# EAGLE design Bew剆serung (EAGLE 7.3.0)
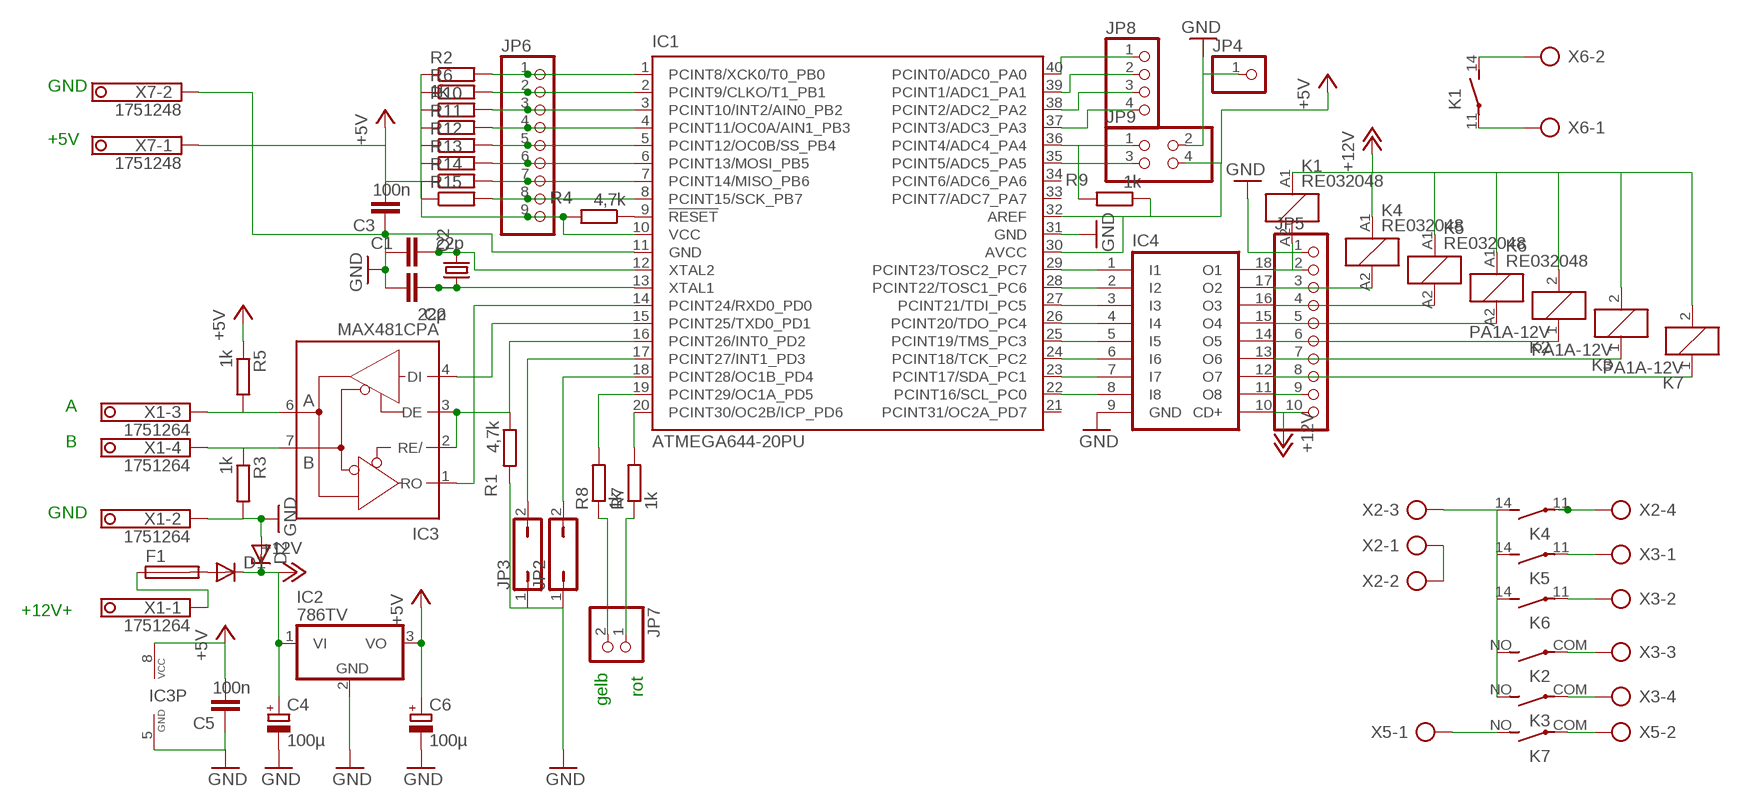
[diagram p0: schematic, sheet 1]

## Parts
C1  22p  C-EUC0603  [C0603]
C2  22p  C-EUC0603  [C0603]
C3  100n  C-EUC1206  [C1206]
C4  100µ  CPOL-EUSMCD  [SMC_D]
C5  100n  C-EU050-024X044  [C050-024X044]
C6  100µ  CPOL-EUSMCD  [SMC_D]
D1  DIODE-DO214AA  [DO214AA]
D2  ZENER-DIODESOD80C  [SOD80C]
F1  19560  [19560]
IC1  ATMEGA644-20PU  [DIL40]
IC2  786TV  [TO220V]
IC3  MAX481CPA  [DIL08]
IC4  ULN2803A  [DIL18]
JP2  JP1Q  [JP1]
JP3  JP1Q  [JP1]
JP4  PINHD-1X1  [1X01]
JP5  PINHD-1X10  [1X10]
JP6  PINHD-1X9  [1X09]
JP7  PINHD-1X2  [1X02]
JP8  PINHD-1X4  [1X04]
JP9  PINHD-2X2  [2X02]
K1  RE032048  [RE-SCHRACK]
K2  PA1A-12V  [PA]
K3  PA1A-12V  [PA]
K4  RE032048  [RE-SCHRACK]
K5  RE032048  [RE-SCHRACK]
K6  RE032048  [RE-SCHRACK]
K7  PA1A-12V  [PA]
Q2  CRYSTALCTS406  [CTS406]
R1  4,7k  R-EU_R0603  [R0603]
R2  1k  R-EU_R0603  [R0603]
R3  1k  R-EU_R1206  [R1206]
R4  4,7k  R-EU_R0603  [R0603]
R5  1k  R-EU_R1206  [R1206]
R6  R-EU_R0603  [R0603]
R7  1k  R-EU_R0603  [R0603]
R8  1k  R-EU_R0603  [R0603]
R9  1k  R-EU_R0603  [R0603]
R10  R-EU_R0603  [R0603]
R11  R-EU_R0603  [R0603]
R12  R-EU_R0603  [R0603]
R13  R-EU_R0603  [R0603]
R14  R-EU_R0603  [R0603]
R15  R-EU_R0603  [R0603]
X1  1751264  [1751264]
X2  AK300/4  [AK300/4]
X3  AK300/4  [AK300/4]
X5  AK300/2  [AK300/2]
X6  AK300/2  [AK300/2]
X7  1751248  [1751248]

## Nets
+5V: C3.2 C5.2 C6.+ IC1.10(VCC) IC1.30(AVCC) IC1.32(AREF) IC2.3(VO) IC3.8(VCC) JP6.9 JP9.4 R2.1 R4.2 R5.1 R6.1 R9.1 R10.1 R11.1 R12.1 R13.1 R14.1 R15.1 X7.1
+12V: C4.+ D1.C D2.C IC2.1(VI) IC4.10(CD+) JP5.10 K1.A1 K2.2 K3.2 K4.A1 K5.A1 K6.A1 K7.2
GND: C1.1 C2.1 C3.1 C4.- C5.1 C6.- D2.A IC1.11(GND) IC1.31(GND) IC2.2(GND) IC3.5(GND) IC4.9(GND) JP2.1 JP3.1 JP4.1 JP5.1 JP9.2 R1.2 R3.2 X1.2 X7.2
N$1: D1.A F1.2
N$2: IC1.14(PCINT24/RXD0_PD0) IC3.1(RO)
N$3: IC3.7(B) R3.1 X1.4
N$4: IC3.6(A) R5.2 X1.3
N$5: IC4.18(O1) JP5.2 K1.A2
N$6: IC1.2(PCINT9/CLKO/T1_PB1) JP6.2 R6.2
N$7: IC1.40(PCINT0/ADC0_PA0) JP8.1
N$8: K4.11(2:P) X2.4
N$9: IC1.29(PCINT23/TOSC2_PC7) IC4.1(I1)
N$10: IC1.15(PCINT25/TXD0_PD1) IC3.4(DI)
N$11: C2.2 IC1.13(XTAL1) Q2.1
N$12: C1.2 IC1.12(XTAL2) Q2.3
N$13: IC1.16(PCINT26/INT0_PD2) IC3.2(RE/) IC3.3(DE) R1.1
N$14: IC1.17(PCINT27/INT1_PD3) JP3.2
N$15: IC1.18(PCINT28/OC1B_PD4) JP2.2
N$16: IC1.28(PCINT22/TOSC1_PC6) IC4.2(I2)
N$17: IC1.27(PCINT21/TDI_PC5) IC4.3(I3)
N$18: IC1.26(PCINT20/TDO_PC4) IC4.4(I4)
N$19: IC1.19(PCINT29/OC1A_PD5) R8.2
N$20: IC1.9(!RESET) R4.1
N$21: IC1.20(PCINT30/OC2B/ICP_PD6) R7.2
N$22: JP7.2 R8.1
N$23: IC1.25(PCINT19/TMS_PC3) IC4.5(I5)
N$24: IC1.24(PCINT18/TCK_PC2) IC4.6(I6)
N$25: JP7.1 R7.1
N$26: IC1.23(PCINT17/SDA_PC1) IC4.7(I7)
N$27: IC1.22(PCINT16/SCL_PC0) IC4.8(I8)
N$28: IC4.17(O2) JP5.3 K4.A2
N$29: IC4.16(O3) JP5.4 K5.A2
N$30: IC4.15(O4) JP5.5 K6.A2
N$31: IC4.14(O5) JP5.6 K2.1
N$32: IC4.13(O6) JP5.7 K3.1
N$33: K1.14(2:S) X6.2
N$34: K1.11(2:P) X6.1
N$35: K2.NO(2:S) K3.NO(2:S) K4.14(2:S) K5.14(2:S) K6.14(2:S) X2.3
N$36: IC1.39(PCINT1/ADC1_PA1) JP8.2
N$37: IC1.38(PCINT2/ADC2_PA2) JP8.3
N$38: IC1.37(PCINT3/ADC3_PA3) JP8.4
N$39: IC1.36(PCINT4/ADC4_PA4) JP9.1 R9.2
N$40: IC1.35(PCINT5/ADC5_PA5) JP9.3
N$41: K5.11(2:P) X3.1
N$42: K6.11(2:P) X3.2
N$43: K2.COM(2:P) X3.3
N$44: K3.COM(2:P) X3.4
N$45: K7.COM(2:P) X5.2
N$46: F1.1 X1.1
N$47: IC1.8(PCINT15/SCK_PB7) JP6.8 R15.2
N$48: IC1.7(PCINT14/MISO_PB6) JP6.7 R14.2
N$49: IC1.6(PCINT13/MOSI_PB5) JP6.6 R13.2
N$50: IC1.5(PCINT12/OC0B/SS_PB4) JP6.5 R12.2
N$51: IC1.4(PCINT11/OC0A/AIN1_PB3) JP6.4 R11.2
N$52: IC1.3(PCINT10/INT2/AIN0_PB2) JP6.3 R10.2
N$53: IC1.1(PCINT8/XCK0/T0_PB0) JP6.1 R2.2
N$54: K7.NO(2:S) X5.1
N$55: IC4.12(O7) JP5.8 K7.1
N$56: IC4.11(O8) JP5.9
N$60: X2.1 X2.2
Unconnected: IC1.21(PCINT31/OC2A_PD7) IC1.33(PCINT7/ADC7_PA7) IC1.34(PCINT6/ADC6_PA6)

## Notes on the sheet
- GND
- +5V
- A
- B
- GND
- +12V+
- rot
- gelb

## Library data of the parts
C1-C3 C5 = rcl:C-EU: CAPACITOR, European symbol
C4 C6 = rcl:CPOL-EU: POLARIZED CAPACITOR, European symbol
D1 = diode:DIODE-: DIODE
D2 = diode:ZENER-DIODE: Z-Diode
F1 = fuse:19560: FUSE HOLDER; MPN: 56000001009; OC_FARNELL: 1185363; OC_NEWARK: 15P8392
IC1 = atmel:ATMEGA644-*PU: 8-bit Microcontroller with 64K Bytes In-System Programmable Flash Auto generated by make-symbol-device-package-bsdl.ulp Rev. 34 Source: http://www.atmel.com/dyn/resources/prod_documents/doc2593.pdf; MPN: ATMEGA644-20PU; OC_FARNELL: 1288340; OC_NEWARK: 23M5060
IC2 = linear:78*: Positive VOLTAGE REGULATOR Source: http://cache.national.com/ds/LM/LM78L05.pdf http://www.fairchildsemi.com/ds/LM/LM7805.pdf
IC3 = maxim:MAX481CPA: RS485 TRANSEIVER; MPN: MAX481CPA+; OC_FARNELL: unknown; OC_NEWARK: 99K3445
IC4 = uln-udn:ULN2803A: DRIVER ARRAY
JP2 JP3 = jumper:JP1Q: JUMPER
JP4 = pinhead:PINHD-1X1: PIN HEADER
JP5 = pinhead:PINHD-1X10: PIN HEADER
JP6 = pinhead:PINHD-1X9: PIN HEADER
JP7 = pinhead:PINHD-1X2: PIN HEADER
JP8 = pinhead:PINHD-1X4: PIN HEADER
JP9 = pinhead:PINHD-2X2: PIN HEADER
K1 K4-K6 = relay:RE03*: Miniature PCB Relay 1 pole 6 A SCHRACK Source: http://www.schrack.com/.. 5812.pdf; OC_FARNELL: unknown; OC_NEWARK: unknown
K2 K3 K7 = relay:PA?*: SLIM POWER RELAY NAiS Source: http://www.mew-europe.com/.. en_ds_61123_0000.pdf; MF: AROMAT/ MATSUSHITA; MPN: PA1A-12V-Y1; OC_FARNELL: 910363; OC_NEWARK: 82H8374
Q2 = crystal:CRYSTAL: CRYSTAL; OC_FARNELL: unknown; OC_NEWARK: unknown
R1-R15 = rcl:R-EU_: RESISTOR, European symbol
X1 = con-phoenix-350:1751264: MKDS 1/ 4-3,5 Printklemme Nennstrom: 10 A Bemessungsspannung: 160 V Raster: 3,5 mm Polzahl: 4 Montageart: Löten Anschlussart: Schraubanschluss Anschlussrichtung vom Leiter zur Platine: 0° Source: http://eshop.phoenixcontact.com .. 1751264.pdf
X2 X3 = con-ptr500:AK300/4: CONNECTOR; OC_FARNELL: unknown; OC_NEWARK: unknown
X5 X6 = con-ptr500:AK300/2: CONNECTOR; OC_FARNELL: unknown; OC_NEWARK: unknown
X7 = con-phoenix-350:1751248: MKDS 1/ 2-3,5 Printklemme

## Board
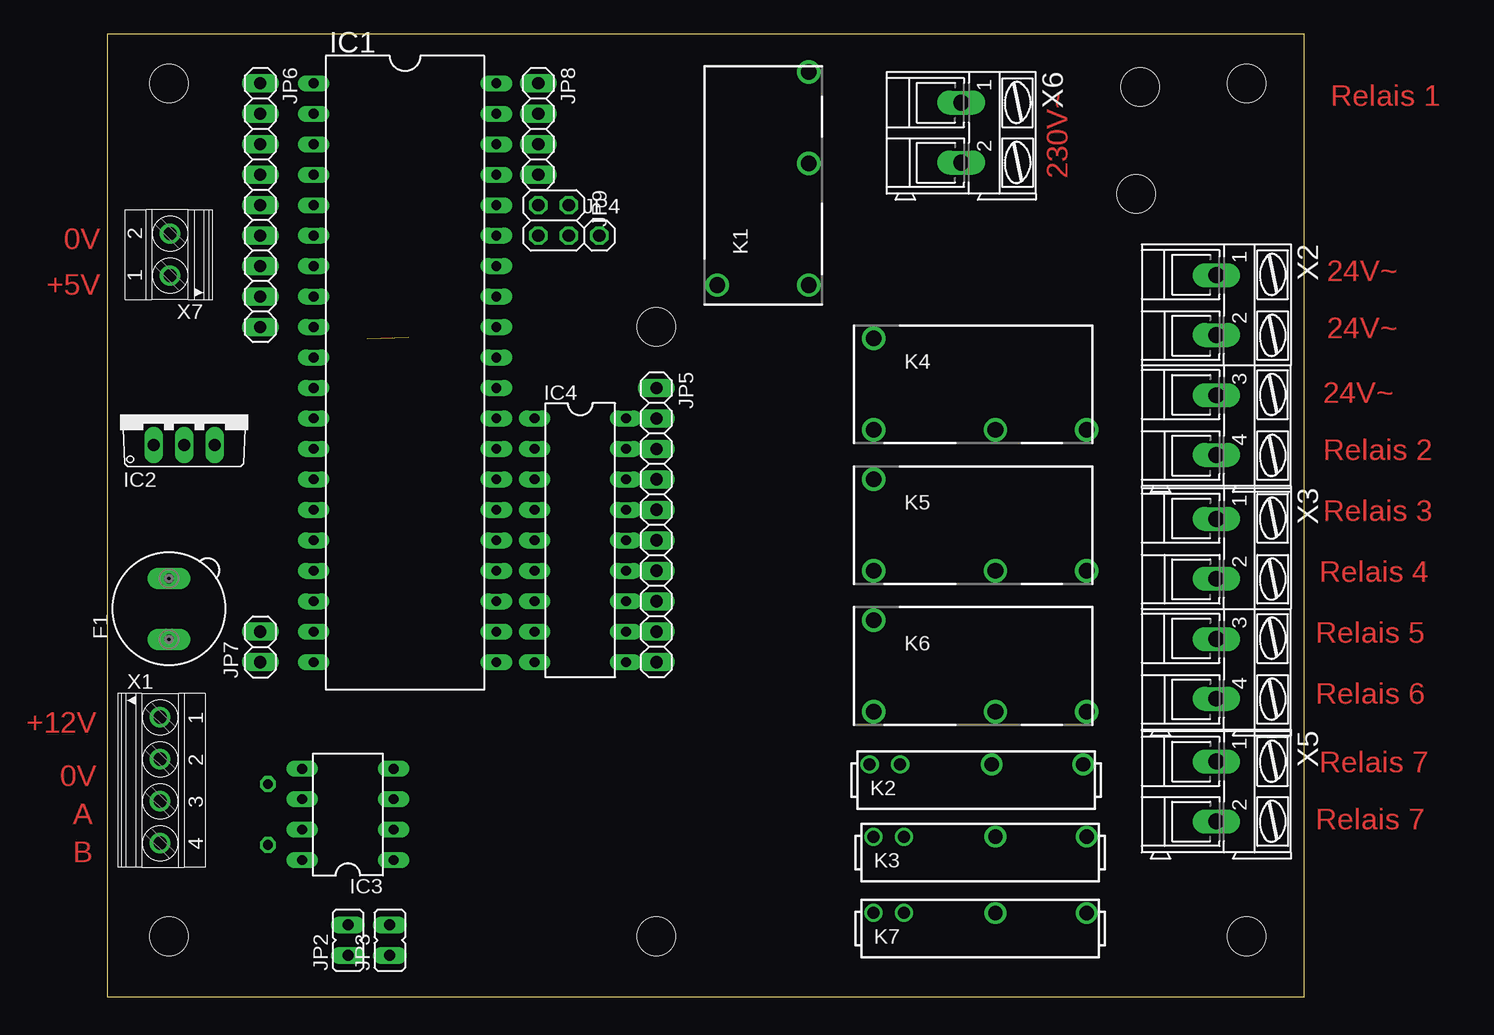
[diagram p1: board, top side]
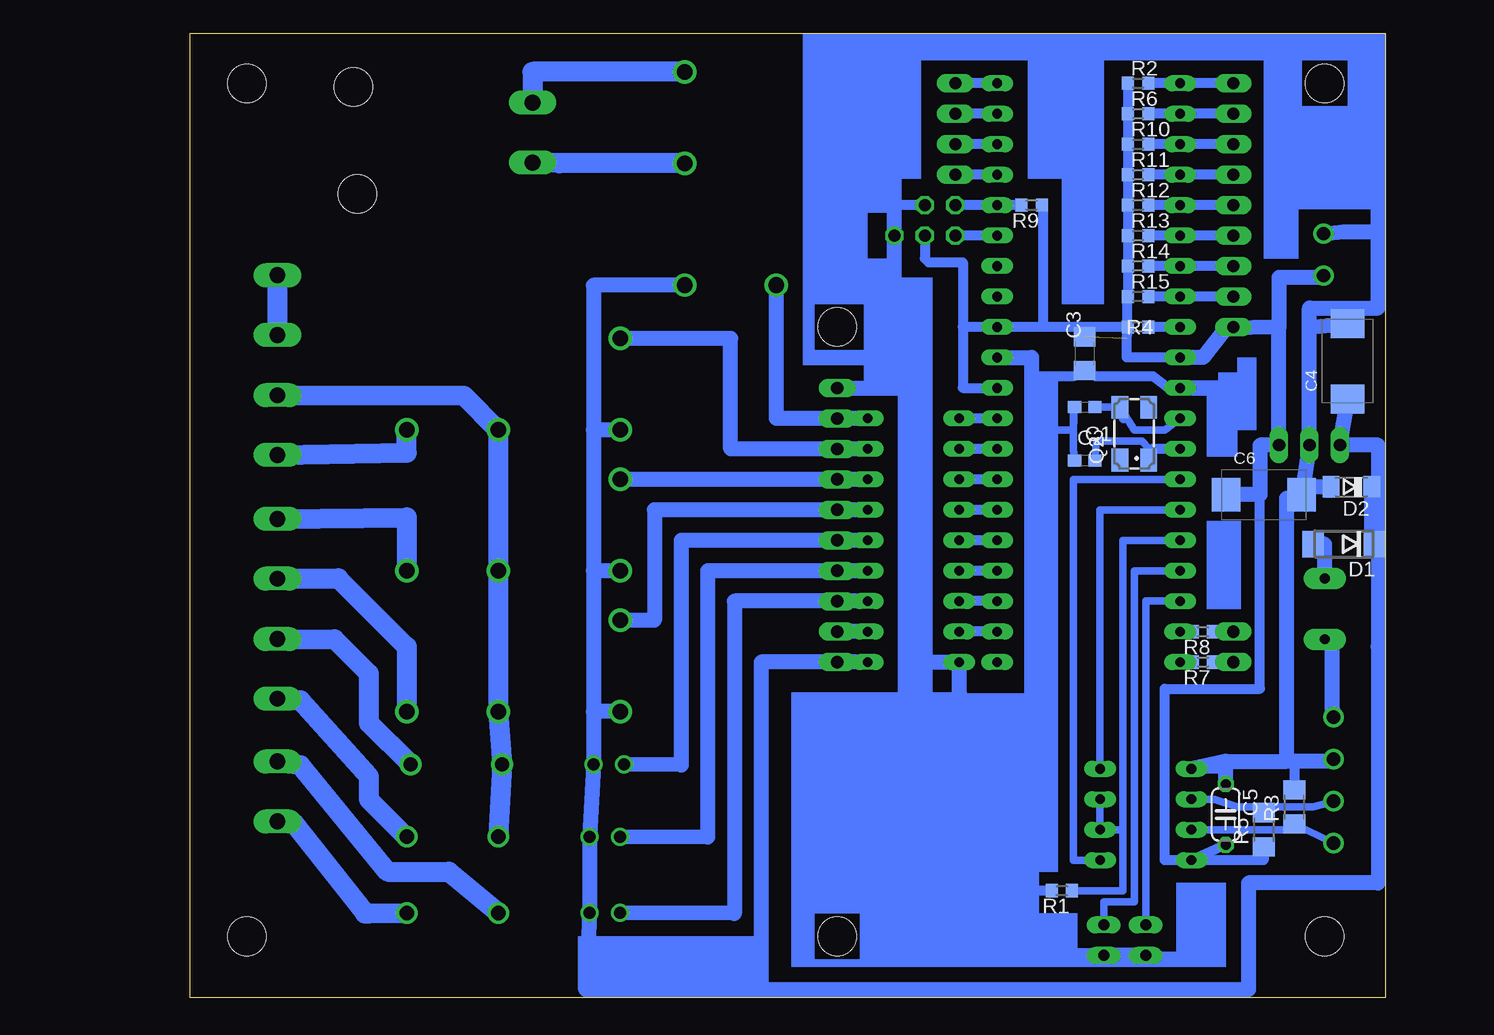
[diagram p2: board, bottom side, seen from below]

Size 99.69 x 80.33 mm. Coordinates in mm from the lower left corner, seen from the top.
Outline: 0,80.33 99.69,80.33 99.69,0 0,0 0,80.33
Copper layers (1*16): Top 0.035mm / dielectric 1.5mm / Bottom 0.035mm
Design rules "default": minimum track width 10mil, minimum drill 24mil, track to track 8mil, track to pad 8mil, pad to pad 8mil, via to via 8mil, smd to smd 8mil, copper to edge 40mil, drill to drill 8mil, minimum pad ring 10mil, minimum via ring 8mil, stop-mask expansion 4mil, vias tented up to drill 0mil, thermal gap 10mil
Holes 3.2 mm at 5.08,76.2 5.08,5.08 94.93,76.2 94.93,5.08 45.72,55.88 45.72,5.08 86.04,75.88 85.72,66.99

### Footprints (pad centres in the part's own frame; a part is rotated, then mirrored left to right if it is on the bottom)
C0603 = smd 1.1 x 1: 1 -0.85,0; 2 0.85,0
C1206 = smd 1.6 x 1.8: 1 -1.4,0; 2 1.4,0
SMC_D = smd 2.4 x 2.8: + -3.15,0; - 3.15,0
C050-024X044 = drill 0.813 octagon: 1 -2.54,0; 2 2.54,0
DO214AA = smd 1.8 x 2.2: A 2.55,0; C -2.55,0
SOD80C = smd 1.4 x 1.8: A 1.7,0; C -1.7,0
19560 = drill 0.813 pad 1.778 long: 1 -2.54,0; 2 2.54,0
DIL40 = drill 0.813 long: 1 -24.13,-7.62; 2 -21.59,-7.62; 3 -19.05,-7.62; 4 -16.51,-7.62; 5 -13.97,-7.62; 6 -11.43,-7.62; 7 -8.89,-7.62; 8 -6.35,-7.62; 9 -3.81,-7.62; 10 -1.27,-7.62; 11 1.27,-7.62; 12 3.81,-7.62; 13 6.35,-7.62; 14 8.89,-7.62; 15 11.43,-7.62; 16 13.97,-7.62; 17 16.51,-7.62; 18 19.05,-7.62; 19 21.59,-7.62; 20 24.13,-7.62; 21 24.13,7.62; 22 21.59,7.62; 23 19.05,7.62; 24 16.51,7.62; 25 13.97,7.62; 26 11.43,7.62; 27 8.89,7.62; 28 6.35,7.62; 29 3.81,7.62; 30 1.27,7.62; 31 -1.27,7.62; 32 -3.81,7.62; 33 -6.35,7.62; 34 -8.89,7.62; 35 -11.43,7.62; 36 -13.97,7.62; 37 -16.51,7.62; 38 -19.05,7.62; 39 -21.59,7.62; 40 -24.13,7.62
TO220V = drill 1.016 long: 1 -2.54,-2.54; 2 0,-2.54; 3 2.54,-2.54
DIL08 = drill 0.813 long: 1 -3.81,-3.81; 2 -1.27,-3.81; 3 1.27,-3.81; 4 3.81,-3.81; 5 3.81,3.81; 6 1.27,3.81; 7 -1.27,3.81; 8 -3.81,3.81
DIL18 = drill 0.813 long: 1 -10.16,-3.81; 2 -7.62,-3.81; 3 -5.08,-3.81; 4 -2.54,-3.81; 5 0,-3.81; 6 2.54,-3.81; 7 5.08,-3.81; 8 7.62,-3.81; 9 10.16,-3.81; 10 10.16,3.81; 11 7.62,3.81; 12 5.08,3.81; 13 2.54,3.81; 14 0,3.81; 15 -2.54,3.81; 16 -5.08,3.81; 17 -7.62,3.81; 18 -10.16,3.81
JP1 = drill 0.914 long: 1 0,-1.27; 2 0,1.27
1X01 = drill 1.016 octagon: 1 0,0
1X10 = drill 1.016 long: 1 -11.43,0; 2 -8.89,0; 3 -6.35,0; 4 -3.81,0; 5 -1.27,0; 6 1.27,0; 7 3.81,0; 8 6.35,0; 9 8.89,0; 10 11.43,0
1X09 = drill 1.016 long: 1 -10.16,0; 2 -7.62,0; 3 -5.08,0; 4 -2.54,0; 5 0,0; 6 2.54,0; 7 5.08,0; 8 7.62,0; 9 10.16,0
1X02 = drill 1.016 long: 1 -1.27,0; 2 1.27,0
1X04 = drill 1.016 long: 1 -3.81,0; 2 -1.27,0; 3 1.27,0; 4 3.81,0
2X02 = drill 1.016 octagon: 1 -1.27,-1.27; 2 -1.27,1.27; 3 1.27,-1.27; 4 1.27,1.27
RE-SCHRACK = drill 1.3: 11 8.89,-3.81; 14 1.27,-3.81; A1 -8.89,-3.81; A2 -8.89,3.81
PA = drill 1: 1 -8.89,1.32; 2 -6.35,1.32 | drill 1.2: COM 8.89,1.32; NO 1.27,1.32
CTS406 = smd 1.9 x 1.4: 1 -2.2,-1.2; 2 2.2,-1.2; 3 2.2,1.2; 4 -2.2,1.2
R0603 = smd 1 x 1.1: 1 -0.85,0; 2 0.85,0
R1206 = smd 1.6 x 1.803: 1 -1.422,0; 2 1.422,0
1751264 = drill 1.1 pad 1.7: 1 -5.25,-0.1; 2 -1.75,-0.1; 3 1.75,-0.1; 4 5.25,-0.1
AK300/4 = drill 1.321 long: 1 -7.493,0; 2 -2.515,0; 3 2.515,0; 4 7.493,0
AK300/2 = drill 1.321 long: 1 -2.515,0; 2 2.489,0
1751248 = drill 1.1 pad 1.7: 1 -1.75,-0.1; 2 1.75,-0.1

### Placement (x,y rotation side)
C1  25.08,49.21 0 bottom
C2  25.08,44.77 0 bottom
C3  25.08,53.66 90 bottom
C4  3.17,53.02 90 bottom
C5  13.34,15.24 270 bottom
C6  10.16,41.91 0 bottom
D1  3.49,37.78 180 bottom
D2  2.86,42.55 180 bottom
F1  5.08,32.38 90 top
IC1  24.77,52.07 270 top
IC2  6.35,48.58 0 top
IC3  20,15.24 90 top
IC4  39.37,38.1 270 top
JP2  20,4.76 0 top
JP3  23.5,4.76 0 top
JP4  40.96,63.5 0 top
JP5  45.72,39.37 270 top
JP6  12.7,66.04 270 top
JP7  12.7,29.21 90 top
JP8  35.88,72.39 270 top
JP9  37.15,64.77 270 top
K1  54.61,68.26 90 top
K2  72.39,18.1 0 top
K3  72.71,12.06 0 top
K4  72.71,51.12 0 top
K5  72.71,39.37 0 top
K6  72.71,27.62 0 top
K7  72.71,5.71 0 top
Q2  20.95,46.99 90 bottom
R1  26.99,8.89 180 bottom
R2  20.64,76.2 0 bottom
R3  7.62,15.88 90 bottom
R4  20.64,55.88 180 bottom
R5  10.16,13.97 90 bottom
R6  20.64,73.66 0 bottom
R7  15.24,27.94 180 bottom
R8  15.24,30.48 180 bottom
R9  29.53,66.04 180 bottom
R10  20.64,71.12 0 bottom
R11  20.64,68.58 0 bottom
R12  20.64,66.04 0 bottom
R13  20.64,63.5 0 bottom
R14  20.64,60.96 0 bottom
R15  20.64,58.42 0 bottom
X1  4.45,18.1 270 top
X2  92.39,52.7 270 top
X3  92.39,32.38 270 top
X5  92.39,17.14 270 top
X6  71.12,72.07 270 top
X7  5.08,61.91 90 top

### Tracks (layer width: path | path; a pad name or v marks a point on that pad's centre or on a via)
+5V  (1 unrouted)
  Bottom 0.813: 35.24,55.88 IC1.32 28.57,55.88 | 35.24,55.88 35.24,50.8 IC1.30 | 35.24,55.88 35.24,61.28 38.1,61.28 38.42,61.59 JP9.4 | 21.59,55.88 R4.2 21.59,54.93 21.59,53.34 IC1.10 | 21.59,55.88 28.57,55.88 | R2.1 R6.1 R10.1 R11.1 R12.1 R13.1 R14.1 R15.1 21.59,58.42 21.59,55.88 | R5.1 10.16,11.43 IC3.8 | IC3.8 18.41,11.43 18.41,25.72 10.48,25.72 10.48,41.91 | C5.2 IC3.8 | R9.1 28.57,66.04 28.57,55.88
  Bottom 1.27: JP6.9 13.33,55.81 | 13.33,55.81 15.24,53.34 IC1.10 | 8.89,55.88 IC2.3 10.48,46.04 10.48,41.91 C6.+ | 8.89,55.88 13.33,55.81 | X7.1 5.71,60.01 8.89,60.01 8.89,55.88
+12V
  Bottom 1.27: JP5.10 IC4.10 52.07,27.94 52.07,0.64 | C4.+ IC2.1 0.64,46.04 0.64,37.78 | 0.64,37.78 0.64,29.21 | 52.07,0.64 66.67,0.64 K7.2 K3.2 K2.2 66.04,23.81 | D1.C 0.64,38.42 | 0.64,38.42 0.64,29.21 | K1.A1 66.04,59.37 66.04,47.31 | 66.04,47.31 66.04,35.56 | 66.04,35.56 66.04,23.81 | K6.A1 66.04,23.81 | K5.A1 66.04,35.56 | K4.A1 66.04,47.31 | 0.64,38.42 0.95,38.42 0.95,37.78 | 0.95,37.78 0.64,37.78 | 0.95,37.78 1.16,37.78 D2.C | 0.64,29.21 0.64,9.53 11.43,9.53 11.43,0.64 52.07,0.64
GND
  Bottom 0.61: 26.04,47.31 26.04,48.58 C1.1 26.04,47.31 | 26.04,47.31 26.04,45.72 C2.1 | 26.04,47.31 29.53,47.31
  Bottom 0.813: IC3.5 13.34,19.01 C5.1 | 7.62,19.68 R3.2 | IC1.11 18.1,50.8 19.37,51.75 24.13,51.75 C3.1 26.04,51.75 29.53,51.75 | R1.2 29.53,8.89 | JP9.2 40.96,66.04 JP4.1
  Bottom 1.27: C6.- IC2.2 6.35,55.88 | 6.35,55.88 C4.- | JP2.1 JP3.1 29.53,3.49 29.53,8.89 29.53,24.77 | X1.2 4.76,19.68 7.62,19.68 8.26,19.68 | 13.34,19.68 IC3.5 | D2.A 6.67,42.55 C6.- | C5.1 13.34,19.68 | 13.34,19.68 8.26,19.68 | 8.26,19.68 8.26,41.59 C6.- | IC1.31 29.53,53.34 29.53,51.75 29.53,47.31 29.53,24.77 | 29.53,24.77 35.56,24.77 IC4.9 39.69,27.94 39.69,50.8 | 39.69,50.8 39.69,59.05 40.96,59.05 40.96,66.04 40.96,78.11 43.18,79.38 0.64,79.38 0.64,63.82 | JP5.1 39.69,50.8 | 6.35,55.88 6.35,57.47 0.64,57.47 0.64,63.82 | X7.2 3.49,63.82 0.64,63.82
N$1
  Bottom 1.27: F1.2 5.08,37.78 D1.A
N$2
  Bottom 0.61: IC3.1 26.04,11.43 26.04,43.18 IC1.14
N$3
  Bottom 0.61: X1.4 R3.1 8.26,13.97 IC3.7
N$4
  Bottom 0.35: R5.2 10.48,15.39 10.48,15.88
  Bottom 0.61: X1.3 6.03,15.88 10.48,15.88 12.38,15.88 14.29,16.51 IC3.6
N$5
  Bottom 1.27: IC4.18 JP5.2 50.8,48.26 K1.A2
N$6
  Bottom 0.813: R6.2 IC1.2 JP6.2
N$7
  Bottom 0.813: IC1.40 JP8.1
N$8
  Bottom 1.676: X2.4 81.6,45.4 K4.11
N$9
  Bottom 0.813: IC1.29 IC4.1
N$10
  Bottom 0.61: IC3.4 23.81,40.64 IC1.15
N$11
  Bottom 0.61: IC1.13 19.68,45.72 20.32,46.35 24.13,46.35 C2.2
  Bottom 0.813: IC1.13 19.44,45.72 Q2.1
N$12
  Bottom 0.61: IC1.12 18.41,47.31 20.95,47.31 Q2.3 C1.2
  Bottom 0.813: 21.84,48.26 Q2.3
N$13
  Bottom 0.61: IC3.3 IC3.2 21.91,13.97 | 21.91,13.97 21.91,38.1 IC1.16 | R1.1 21.91,8.89 21.91,13.97
N$14
  Bottom 0.61: IC1.17 20.95,35.56 20.95,7.94 23.5,7.94 JP3.2
N$15
  Bottom 0.61: IC1.18 20,33.02 JP2.2
N$16
  Bottom 0.813: IC1.28 IC4.2
N$17
  Bottom 0.813: IC1.27 IC4.3
N$18
  Bottom 0.813: IC1.26 IC4.4
N$19
  Bottom 0.813: R8.2 IC1.19
N$20
  Bottom 0.813: IC1.9 R4.1
N$21
  Bottom 0.813: R7.2 IC1.20
N$22
  Bottom 0.813: JP7.2 R8.1
N$23
  Bottom 0.813: IC1.25 IC4.5
N$24
  Bottom 0.813: IC1.24 IC4.6
N$25
  Bottom 0.813: JP7.1 R7.1
N$26
  Bottom 0.813: IC1.23 IC4.7
N$27
  Bottom 0.813: IC1.22 IC4.8
N$28
  Bottom 1.27: IC4.17 JP5.3 54.61,45.72 54.61,54.93 K4.A2
N$29
  Bottom 1.27: IC4.16 JP5.4 K5.A2
N$30
  Bottom 1.27: IC4.15 JP5.5 60.96,40.64 60.96,31.43 K6.A2
N$31
  Bottom 1.27: IC4.14 JP5.6 58.74,38.1 58.74,19.37 K2.1
N$32
  Bottom 1.27: IC4.13 JP5.7 56.52,35.56 56.52,13.34 K3.1
N$33
  Bottom 1.676: K1.14 68.9,69.53 X6.2
N$34
  Bottom 1.676: K1.11 71.12,77.15 X6.1
N$35
  Bottom 1.676: K3.NO K2.NO K6.14 K5.14 K4.14 76.83,50.16 X2.3
N$36
  Bottom 0.813: IC1.39 JP8.2
N$37
  Bottom 0.813: IC1.38 JP8.3
N$38
  Bottom 0.813: IC1.37 JP8.4
N$39
  Bottom 0.813: JP9.1 IC1.36 R9.2
N$40
  Bottom 0.813: IC1.35 JP9.3
N$41
  Bottom 1.676: X3.1 81.6,40.01 K5.11
N$42
  Bottom 1.676: X3.2 87.31,34.92 81.6,29.21 K6.11
N$43
  Bottom 1.676: X3.3 87.63,29.84 84.77,26.99 84.77,22.86 K2.COM
N$44
  Bottom 1.676: X3.4 90.49,24.77 84.77,18.41 84.77,16.51 81.6,13.34 K3.COM
N$45
  Bottom 1.676: 84.77,6.99 K7.COM 85.09,6.99 91.12,14.61 X5.2
N$46
  Bottom 1.27: X1.1 4.45,23.98 4.45,29.84 F1.1
N$47
  Bottom 0.813: R15.2 IC1.8 JP6.8
N$48
  Bottom 0.813: R14.2 IC1.7 JP6.7
N$49
  Bottom 0.813: R13.2 IC1.6 JP6.6
N$50
  Bottom 0.813: R12.2 IC1.5 JP6.5
N$51
  Bottom 0.813: R11.2 IC1.4 JP6.4
N$52
  Bottom 0.813: R10.2 IC1.3 JP6.3
N$53
  Bottom 0.813: R2.2 IC1.1 JP6.1
N$54
  Bottom 1.676: X5.1 90.49,19.37 83.19,10.48 78.11,10.48 K7.NO
N$55
  Bottom 1.27: IC4.12 JP5.8 54.29,33.02 54.29,6.99 K7.1
N$56
  Bottom 1.27: IC4.11 JP5.9
N$60
  Bottom 1.676: X2.1 X2.2
(copper drawn outside any net)
  shapes: Bottom area x38

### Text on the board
Top: Relais 1 | 230V~ | 0V | +5V | 24V~ | 24V~ | 24V~ | Relais 2 | Relais 3 | Relais 4 | Relais 5 | +12V | Relais 6 | 0V | Relais 7 | A | Relais 7 | B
